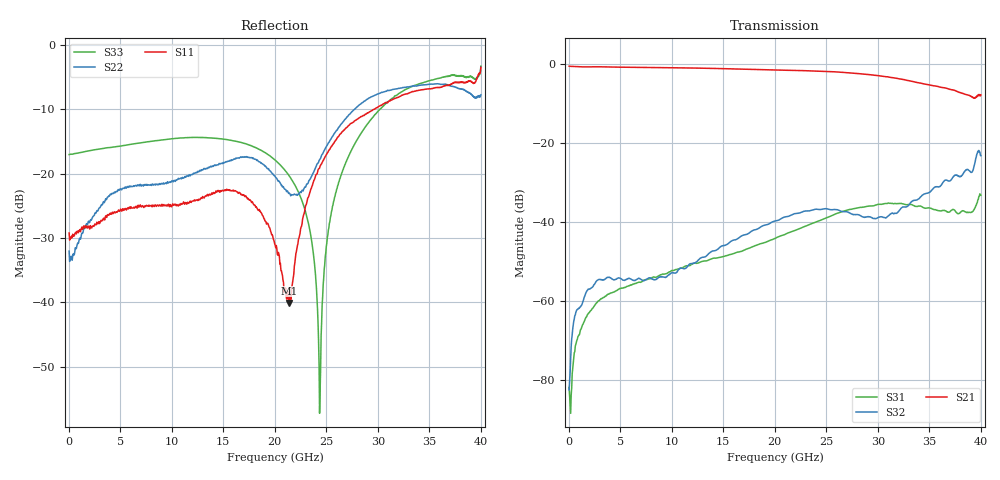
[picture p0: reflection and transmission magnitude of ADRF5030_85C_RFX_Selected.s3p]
! Device  : ADRF5030
! Description: Silicon SPDT Switch Non-Reflective
! Frequency:  100 MHz -  20 GHz
! Ports:
!  RFC = Port 1
!  RF1 = Port 2
!  RF2 = Port 3
! VSS  =  -3.30 Volts
! VDD  =  +3.30 Volts
! EN  =  0.00 Volts
! LS  =  0.00 Volts
! V1  =  +3.30 Volts
! Data:  Data was collected using an calibrated 4 port network analyzer.
! Notes: Analog Devices supplies this data as a sample of measured data
!  for this product.  Your particular data for this product may vary.
!  Data was taken at +85 degrees C.
!  Analog Devices reserves the right to change this data at anytime.
# HZ S DB R 50
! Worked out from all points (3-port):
!   800 points, 50 MHz to 40 GHz, reference 50 ohm
!   strongest paths, dB at 50 MHz, 10.05 GHz, 20.05 GHz, 30.05 GHz, 40 GHz:
!     S21: -0.5, -0.9, -1.5, -2.9, -7.8
!     S32: -82.5, -52.8, -39.7, -38.8, -23.2
!     S31: -81.9, -52.3, -44.1, -35.5, -33.2
!   lowest |S11| = -40.1 dB at 21.4 GHz (marker M1), VSWR 1.02, Z = 49.3 + j0.668 ohm
!   |S11| at or under -10 dB: start of sweep to 29.66 GHz
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5e7  -29.22 -3.6  -0.49 -0.3  -81.86 -14.6
     -0.49 -0.3  -32.05 -9.7  -82.48 10.9
     -81.86 -14.6  -82.48 10.9  -17.04 0.0
1.85e9  -28.40 -63.9  -0.67 -24.2  -63.40 80.5
        -0.67 -24.2  -27.82 -78.0  -57.22 47.6
        -63.40 80.5  -57.22 47.6  -16.49 -19.4
7.8e9  -25.00 146.9  -0.83 -101.4  -54.37 56.6
       -0.83 -101.4  -21.75 -145.9  -54.11 -0.9
       -54.37 56.6  -54.11 -0.9  -15.03 -83.3
1.395e10  -23.20 4.6  -1.06 179.1  -49.21 39.1
          -1.06 179.1  -18.81 -159.7  -47.33 -22.4
          -49.21 39.1  -47.33 -22.4  -14.49 -136.6
2.005e10  -31.14 -122.0  -1.46 96.4  -44.12 -0.5
          -1.46 96.4  -20.45 161.8  -39.68 -66.5
          -44.12 -0.5  -39.68 -66.5  -17.92 172.7
2.14e10  -40.09 136.8  -1.55 77.1  -42.65 -17.8
         -1.55 77.1  -23.02 174.4  -38.46 -77.9
         -42.65 -17.8  -38.46 -77.9  -20.34 161.8
2.435e10  -19.13 21.3  -1.75 33.7  -39.63 -63.0
          -1.75 33.7  -17.84 -143.9  -36.81 -112.7
          -39.63 -63.0  -36.81 -112.7  -57.22 167.9
2.79e10  -11.65 -40.6  -2.34 -17.4  -36.48 -125.7
         -2.34 -17.4  -9.75 -173.9  -38.09 -173.2
         -36.48 -125.7  -38.09 -173.2  -14.98 -86.5
3.635e10  -6.42 -152.3  -5.94 -126.5  -37.02 128.5
          -5.94 -126.5  -6.12 67.6  -29.85 4.7
          -37.02 128.5  -29.85 4.7  -5.00 155.8
4e10  -3.50 80.3  -7.78 128.7  -33.17 83.7
      -7.78 128.7  -7.76 -73.8  -23.18 -117.2
      -33.17 83.7  -23.18 -117.2  -3.32 15.1
